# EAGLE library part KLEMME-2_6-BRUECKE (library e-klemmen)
Klemme 6-pol. mit Brückenhinweis
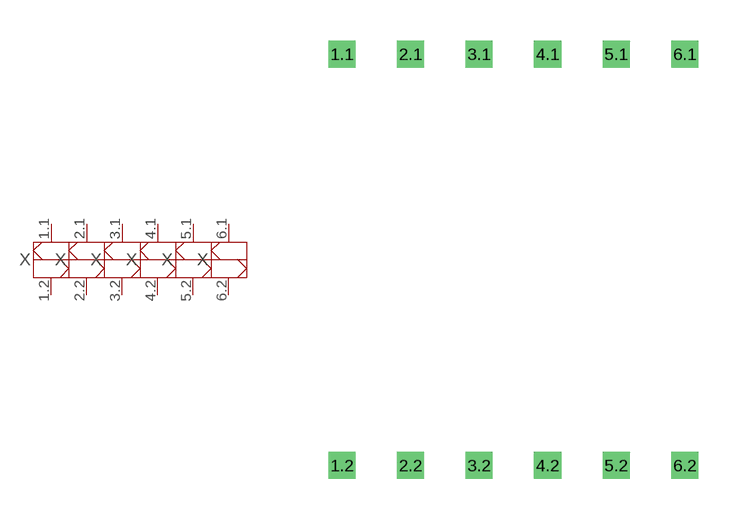
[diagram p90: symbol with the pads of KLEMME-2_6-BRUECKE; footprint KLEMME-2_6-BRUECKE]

Designator prefix X; gates 1=KLEMME-2_1-BRUECKE 2=KLEMME-2_2-BRUECKE 3=KLEMME-2_3-BRUECKE 4=KLEMME-2_4-BRUECKE 5=KLEMME-2_5-BRUECKE 6=KLEMME-2_6-BRUECKE

## KLEMME-2_6-BRUECKE  [KLEMME-2_6-BRUECKE]
1.1  1:1  pas
1.2  1:2  pas
2.1  2:1  pas
2.2  2:2  pas
3.1  3:1  pas
3.2  3:2  pas
4.1  4:1  pas
4.2  4:2  pas
5.1  5:1  pas
5.2  5:2  pas
6.1  6:1  pas
6.2  6:2  pas

## Footprint KLEMME-2_6-BRUECKE (pad centres in mm)
Dummy
drill 0.5 pad 1 square: 1.1 0,0; 1.2 0,-15.24; 2.1 2.54,0; 2.2 2.54,-15.24; 3.1 5.08,0; 3.2 5.08,-15.24; 4.1 7.62,0; 4.2 7.62,-15.24; 5.1 10.16,0; 5.2 10.16,-15.24; 6.1 12.7,0; 6.2 12.7,-15.24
